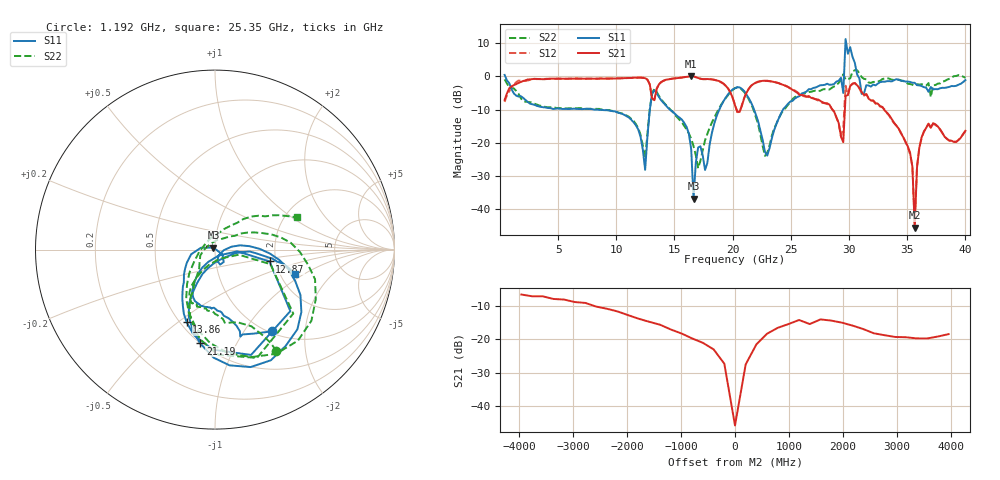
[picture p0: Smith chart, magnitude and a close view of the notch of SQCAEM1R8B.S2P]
! Network Analyzer HP8722ES.07.66: Jul 25, 2000 Serial No. US39175408
! 26 Oct 2004  11:02:42
! Frequency  S11  S21  S12  S22
# HZ  S  DB R  50
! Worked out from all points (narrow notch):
!   201 points, 400 MHz to 40 GHz, reference 50 ohm
!   highest |S21| = 0.06 dB at 16.44 GHz (marker M1); lowest = -45.7 dB at 35.64 GHz (marker M2)
!   notch at M2: 43.4 dB deep, 666 MHz wide at half that depth
!   lowest |S11| = -37.0 dB at 16.64 GHz (marker M3), VSWR 1.03, Z = 49.1 + j1.12 ohm
!   |S11| at or under -10 dB: 8.337 GHz to 12.88 GHz (4.542 GHz wide, 42.8 % of centre); 14.61 GHz to 18.85 GHz (4.246 GHz wide, 25.4 % of centre); 21.84 GHz to 24.33 GHz (2.494 GHz wide, 10.8 % of centre)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
!   |S22| runs from -27.7 to 1.9 dB; largest |S21 - S12| = 0.28
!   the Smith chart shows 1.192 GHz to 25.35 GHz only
!   S11 on the Smith chart (normalised r, x): 1.192 GHz: 1.03, -1.36; 12.87 GHz: 1.85, -0.27; 13.86 GHz: 0.54, -0.54; 21.19 GHz: 0.50, -0.72; 25.35 GHz: 2.40, -0.83
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4e8  0.47 -25.1  -7.09 66.0  -7.67 71.4  -0.86 -16.9
1.192e9  -5.11 -55.0  -2.62 34.9  -2.51 30.1  -3.61 -58.8
7.132e9  -9.86 -103.2  -0.66 -14.9  -0.70 -15.4  -9.75 -108.1
1.2874e10  -10.14 -12.3  -2.33 -64.2  -2.41 -64.6  -9.92 -14.7
1.3666e10  -6.20 -104.1  -2.35 -21.6  -2.27 -21.3  -5.89 -99.3
1.3864e10  -7.24 -111.2  -1.69 -25.2  -1.64 -25.0  -6.93 -105.0
1.6438e10  -22.06 172.5  0.06 -51.1  0.10 -50.8  -18.83 -138.8
1.6636e10  -36.96 126.8  0.01 -54.5  0.07 -54.0  -21.05 -157.8
2.02e10  -3.54 -53.7  -8.70 -92.3  -8.67 -91.6  -3.51 -36.4
2.119e10  -5.52 -99.0  -4.88 -36.5  -4.87 -36.7  -5.66 -93.0
2.5348e10  -6.66 -16.8  -4.47 -98.1  -4.25 -98.6  -6.23 21.5
2.6932e10  -3.46 -34.3  -6.64 -98.2  -6.60 -98.5  -4.40 5.4
2.9506e10  -4.98 25.1  -19.86 -160.7  -15.52 -134.0  0.69 28.9
2.9704e10  11.31 -55.9  -5.93 -61.3  -2.79 -44.3  -0.96 -57.7
3.0496e10  4.16 -81.8  -1.96 -67.7  -2.02 -67.0  1.90 -22.0
3.0694e10  0.62 88.1  -2.64 -85.9  -2.67 -85.0  1.89 145.3
3.1288e10  -5.05 120.9  -5.61 -98.6  -5.79 -100.5  -0.72 137.1
3.1486e10  -2.63 -54.2  -5.30 -95.9  -5.40 -97.6  -0.85 -39.2
3.3466e10  -1.41 -41.9  -11.74 -114.0  -11.94 -114.5  -0.66 -31.2
3.5644e10  -1.90 -64.8  -45.69 -87.7  -44.40 -82.4  -2.85 -18.9
3.6436e10  -3.22 -68.2  -16.62 -8.7  -16.68 -9.9  -2.54 -13.6
4e10  -1.08 -61.7  -16.42 -22.8  -16.50 -22.2  -0.37 -18.2
